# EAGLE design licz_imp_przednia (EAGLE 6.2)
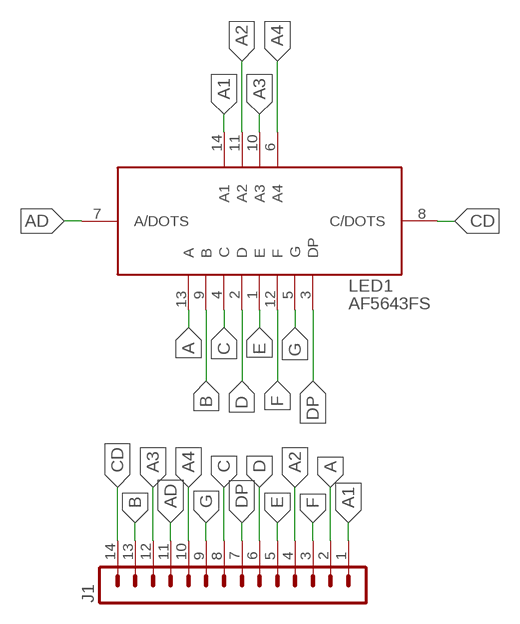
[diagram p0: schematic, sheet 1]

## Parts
J1  MA14-1  [MA14-1]
LED1  AF5643FS  LED_DISP_AF5643FS  [LED_DISP_AF5643FS]

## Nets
A: J1.2 LED1.13(A)
A1: J1.1 LED1.14(A1)
A2: J1.4 LED1.11(A2)
A3: J1.12 LED1.10(A3)
A4: J1.10 LED1.6(A4)
AD: J1.11 LED1.7(A/DOTS)
B: J1.13 LED1.9(B)
C: J1.8 LED1.4(C)
CD: J1.14 LED1.8(C/DOTS)
D: J1.6 LED1.2(D)
DP: J1.7 LED1.3(DP)
E: J1.5 LED1.1(E)
F: J1.3 LED1.12(F)
G: J1.9 LED1.5(G)

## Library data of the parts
J1 = zlacza_futrzak:MA14-1: PIN HEADER; OC_FARNELL: unknown; OC_NEWARK: unknown
LED1 = inne_futrzak:LED_DISP_AF5643FS

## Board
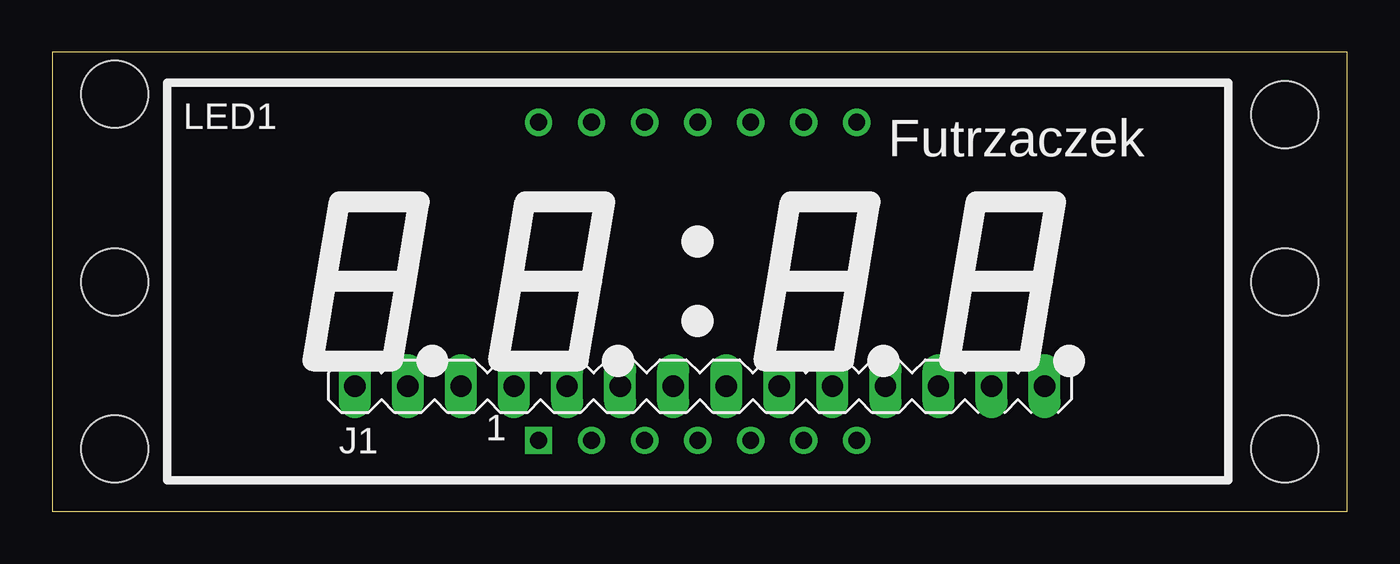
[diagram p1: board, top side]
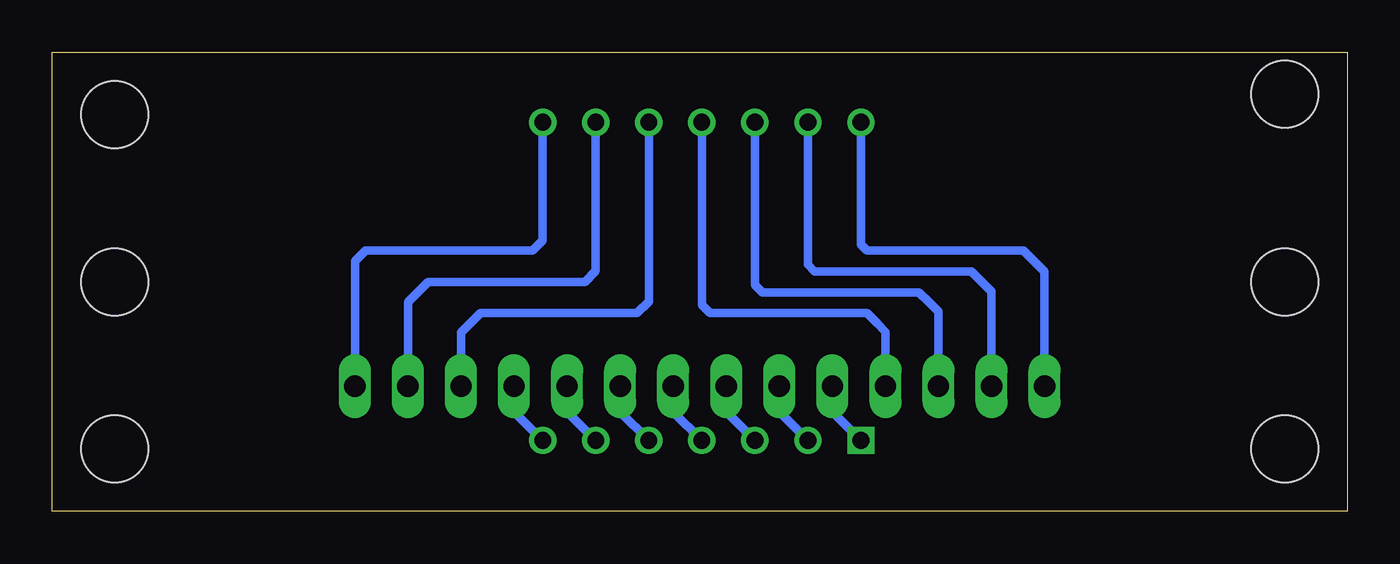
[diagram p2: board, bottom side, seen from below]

Size 62 x 22 mm. Coordinates in mm from the lower left corner, seen from the top.
Outline: 0,0 62,0 62,22 0,22 0,0
Copper layers (1*16): Top 0.035mm / dielectric 1.5mm / Bottom 0.035mm
Design rules: minimum track width 10mil, minimum drill 24mil, track to track 8mil, track to pad 8mil, pad to pad 8mil, via to via 8mil, smd to smd 8mil, copper to edge 40mil, drill to drill 8mil, minimum pad ring 10mil, minimum via ring 8mil, stop-mask expansion 4mil, vias tented up to drill 0mil, thermal gap 10mil
Holes 3.2 mm at 3,3 3,11 3,20 59,3 59,11 59,19

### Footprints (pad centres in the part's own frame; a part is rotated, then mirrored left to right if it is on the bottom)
MA14-1 = drill 1.016 long: 1 -16.51,0; 2 -13.97,0; 3 -11.43,0; 4 -8.89,0; 5 -6.35,0; 6 -3.81,0; 7 -1.27,0; 8 1.27,0; 9 3.81,0; 10 6.35,0; 11 8.89,0; 12 11.43,0; 13 13.97,0; 14 16.51,0
LED_DISP_AF5643FS = drill 0.8 square: 1 17.78,1.905 | drill 0.8: 2 20.32,1.905; 3 22.86,1.905; 4 25.4,1.905; 5 27.94,1.905; 6 30.48,1.905; 7 33.02,1.905; 8 33.02,17.145; 9 30.48,17.145; 10 27.94,17.145; 11 25.4,17.145; 12 22.86,17.145; 13 20.32,17.145; 14 17.78,17.145

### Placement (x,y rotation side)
J1  31,6 0 top
LED1  5.5,1.5 0 top

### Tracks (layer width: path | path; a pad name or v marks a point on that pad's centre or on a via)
A
  Bottom 0.406: LED1.13 25.82,11.82 25.5,11.5 18,11.5 17.5,11 17.03,10.53 J1.2
A1
  Bottom 0.406: LED1.14 23.28,12.78 23,12.5 15.5,12.5 15,12 14.49,11.49 J1.1
A2
  Bottom 0.406: LED1.11 30.9,9.9 30.5,9.5 23,9.5 22.5,9 22.11,8.61 J1.4
A3
  Bottom 0.406: LED1.10 33.44,10.06 34,9.5 41.5,9.5 42,9 42.43,8.57 J1.12
A4
  Bottom 0.406: J1.10 37.35,4.78 LED1.6
AD
  Bottom 0.406: J1.11 39.89,4.78 LED1.7
B
  Bottom 0.406: LED1.9 35.98,11.52 36.5,11 44,11 44.5,10.5 44.97,10.03 J1.13
C
  Bottom 0.406: J1.8 32.27,4.78 LED1.4
CD
  Bottom 0.406: LED1.8 38.52,12.98 39,12.5 47,12.5 47.51,11.99 J1.14
D
  Bottom 0.406: J1.6 27.19,4.78 LED1.2
DP
  Bottom 0.406: J1.7 29.73,4.78 LED1.3
E
  Bottom 0.406: J1.5 24.65,4.78 LED1.1
F
  Bottom 0.406: LED1.12 28.36,10.86 28,10.5 20.5,10.5 20,10 19.57,9.57 J1.3
G
  Bottom 0.406: J1.9 34.81,4.78 LED1.5

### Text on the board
tPlace: Futrzaczek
